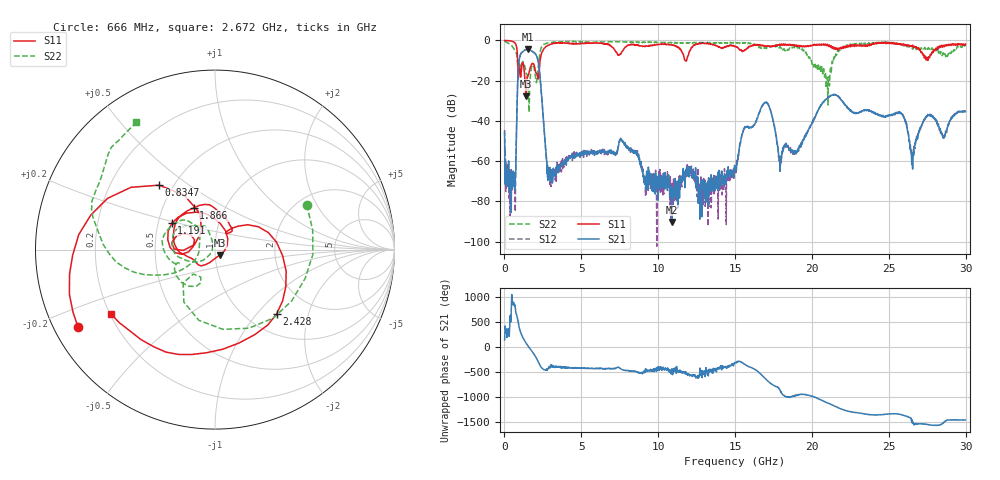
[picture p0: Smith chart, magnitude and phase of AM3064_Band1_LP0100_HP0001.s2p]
# Hz S DB R 50.0
!freq dBS11 angS11 dBS21 angS21 dBS12 angS12 dBS22 angS22
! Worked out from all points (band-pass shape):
!   1600 points, 10 MHz to 29.98 GHz, reference 50 ohm
!   highest |S21| = -4.50 dB at 1.51 GHz (marker M1); lowest = -90.2 dB at 10.9 GHz (marker M2)
!   |S21| within 3 dB of the highest: 1.024 GHz to 2.074 GHz (1.05 GHz wide, 67.8 % of centre)
!   lowest |S11| = -27.8 dB at 1.397 GHz (marker M3), VSWR 1.08, Z = 52.8 - j3.15 ohm
!   |S11| at or under -10 dB: 857.3 MHz to 2.318 GHz (1.461 GHz wide, 92 % of centre); 11.75 GHz to 11.84 GHz (89.96 MHz wide, 0.763 % of centre)
!   |S22| runs from -35.7 to -0.4 dB; largest |S21 - S12| = 0.0074
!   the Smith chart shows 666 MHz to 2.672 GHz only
!   S11 on the Smith chart (normalised r, x): 666 MHz: 0.07, -0.26; 834.7 MHz: 0.42, +0.39; 1.191 GHz: 0.59, +0.19; 1.866 GHz: 0.71, +0.36; 2.428 GHz: 1.35, -1.28; 2.672 GHz: 0.20, -0.27
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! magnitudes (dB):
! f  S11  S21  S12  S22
! 10 MHz  0.0  -45.7  -44.6  -0.4
! 666 MHz  -1.1  -74.5  -70.1  -4.9
! 834.7 MHz  -6.5  -27.6  -27.5  -9.4
! 1.191 GHz  -11.0  -5.7  -5.6  -10.5
! 1.397 GHz  -27.8  -4.6  -4.5  -15.9
! 1.51 GHz  -17.9  -4.5  -4.5  -19.4
! 1.866 GHz  -11.7  -5.8  -5.8  -12.2
! 2.428 GHz  -6.1  -29.0  -28.9  -3.1
! 2.672 GHz  -3.3  -53.6  -53.1  -1.6
! 2.953 GHz  -2.1  -63.1  -71.7  -1.1
! 5.015 GHz  -1.5  -57.2  -55.3  -0.7
! 7.639 GHz  -5.6  -49.8  -49.7  -0.7
! 10 GHz  -2.0  -79.4  -69.6  -1.0
! 10.9 GHz  -2.3  -90.2  -77.6  -1.1
! 15 GHz  -3.1  -64.6  -63.2  -1.4
! 16.92 GHz  -2.8  -30.9  -30.9  -3.9
! 17.97 GHz  -2.4  -60.8  -60.1  -3.4
! 19.99 GHz  -2.7  -41.3  -41.2  -11.1
! 21.42 GHz  -3.8  -27.0  -26.9  -8.8
! 25 GHz  -1.0  -37.2  -37.4  -1.2
! 26.53 GHz  -2.4  -61.2  -58.2  -4.3
! 29.98 GHz  -1.9  -35.5  -35.5  -2.9
